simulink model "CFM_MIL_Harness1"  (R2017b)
settings: Solver=FixedStepDiscrete  StartTime=0.0  StopTime=14  FixedStep=0.01  RelTol=1e-3  EnableMultiTasking=on
undefined symbols (not defined in the file): sigbuilder_block
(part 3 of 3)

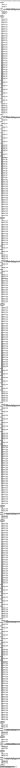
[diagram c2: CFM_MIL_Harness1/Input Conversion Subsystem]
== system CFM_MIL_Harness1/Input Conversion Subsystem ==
  note: This subsystem has been inserted by Simulink to adapt the output of the source blocks to the interface required by the harnessed component. Modifying the contents of this subsystem may result in compilation and simulation failure.
  Inport_1 : Inport
  Inport_2 : Inport  Port=2
  Inport_3 : Inport  Port=3
  Inport_4 : Inport  Port=4
  Inport_5 : Inport  Port=5
  Inport_6 : Inport  Port=6
  Inport_7 : Inport  Port=7
  Inport_8 : Inport  Port=8
  Inport_9 : Inport  Port=9
  Inport_10 : Inport  Port=10
  Inport_11 : Inport  Port=11
  Inport_12 : Inport  Port=12
  Inport_13 : Inport  Port=13
  Inport_14 : Inport  Port=14
  Inport_15 : Inport  Port=15
  Inport_16 : Inport  Port=16
  Inport_17 : Inport  Port=17
  Inport_18 : Inport  Port=18
  Inport_19 : Inport  Port=19
  Inport_20 : Inport  Port=20
  Inport_21 : Inport  Port=21
  Inport_22 : Inport  Port=22
  Inport_23 : Inport  Port=23
  Inport_24 : Inport  Port=24
  Inport_25 : Inport  Port=25
  Inport_26 : Inport  Port=26
  Inport_27 : Inport  Port=27
  Inport_28 : Inport  Port=28
  Inport_29 : Inport  Port=29
  Inport_30 : Inport  Port=30
  Inport_31 : Inport  Port=31
  Inport_32 : Inport  Port=32
  Inport_33 : Inport  Port=33
  Inport_34 : Inport  Port=34
  Inport_35 : Inport  Port=35
  Inport_36 : Inport  Port=36
  Inport_37 : Inport  Port=37
  Inport_38 : Inport  Port=38
  Inport_39 : Inport  Port=39
  Inport_40 : Inport  Port=40
  Inport_41 : Inport  Port=41
  Inport_42 : Inport  Port=42
  Inport_43 : Inport  Port=43
  Inport_44 : Inport  Port=44
  Inport_45 : Inport  Port=45
  Inport_46 : Inport  Port=46
  Inport_47 : Inport  Port=47
  Inport_48 : Inport  Port=48
  Inport_49 : Inport  Port=49
  Inport_50 : Inport  Port=50
  Inport_51 : Inport  Port=51
  Inport_52 : Inport  Port=52
  Inport_53 : Inport  Port=53
  Inport_54 : Inport  Port=54
  Inport_55 : Inport  Port=55
  Inport_56 : Inport  Port=56
  Inport_57 : Inport  Port=57
  Inport_58 : Inport  Port=58
  Inport_59 : Inport  Port=59
  Inport_60 : Inport  Port=60
  Inport_61 : Inport  Port=61
  Inport_62 : Inport  Port=62
  Inport_63 : Inport  Port=63
  Inport_64 : Inport  Port=64
  Inport_65 : Inport  Port=65
  Inport_66 : Inport  Port=66
  Inport_67 : Inport  Port=67
  Inport_68 : Inport  Port=68
  Inport_69 : Inport  Port=69
  Inport_70 : Inport  Port=70
  Inport_71 : Inport  Port=71
  Inport_72 : Inport  Port=72
  Inport_73 : Inport  Port=73
  Inport_74 : Inport  Port=74
  Inport_75 : Inport  Port=75
  Inport_76 : Inport  Port=76
  Inport_77 : Inport  Port=77
  Inport_78 : Inport  Port=78
  Inport_79 : Inport  Port=79
  Inport_80 : Inport  Port=80
  Inport_81 : Inport  Port=81
  Inport_82 : Inport  Port=82
  Inport_83 : Inport  Port=83
  Inport_84 : Inport  Port=84
  Inport_85 : Inport  Port=85
  Inport_86 : Inport  Port=86
  Inport_87 : Inport  Port=87
  Inport_88 : Inport  Port=88
  Inport_89 : Inport  Port=89
  Inport_90 : Inport  Port=90
  Inport_91 : Inport  Port=91
  Inport_92 : Inport  Port=92
  Inport_93 : Inport  Port=93
  Inport_94 : Inport  Port=94
  Inport_95 : Inport  Port=95
  Inport_96 : Inport  Port=96
  Inport_97 : Inport  Port=97
  Inport_98 : Inport  Port=98
  Inport_99 : Inport  Port=99
  Inport_100 : Inport  Port=100
  Inport_101 : Inport  Port=101
  Inport_102 : Inport  Port=102
  Inport_103 : Inport  Port=103
  Inport_104 : Inport  Port=104
  Inport_105 : Inport  Port=105
  Inport_106 : Inport  Port=106
  Inport_107 : Inport  Port=107
  Inport_108 : Inport  Port=108
  Inport_109 : Inport  Port=109
  Inport_110 : Inport  Port=110
  Inport_111 : Inport  Port=111
  Inport_112 : Inport  Port=112
  Inport_113 : Inport  Port=113
  Inport_114 : Inport  Port=114
  Inport_115 : Inport  Port=115
  Inport_116 : Inport  Port=116
  Inport_117 : Inport  Port=117
  Inport_118 : Inport  Port=118
  Inport_119 : Inport  Port=119
  Inport_120 : Inport  Port=120
  Inport_121 : Inport  Port=121
  Inport_122 : Inport  Port=122
  Inport_123 : Inport  Port=123
  Inport_124 : Inport  Port=124
  Inport_125 : Inport  Port=125
  Inport_126 : Inport  Port=126
  Inport_127 : Inport  Port=127
  Inport_128 : Inport  Port=128
  Inport_129 : Inport  Port=129
  Inport_130 : Inport  Port=130
  Inport_131 : Inport  Port=131
  Inport_132 : Inport  Port=132
  Inport_133 : Inport  Port=133
  Inport_134 : Inport  Port=134
  Inport_135 : Inport  Port=135
  Inport_136 : Inport  Port=136
  Inport_137 : Inport  Port=137
  Inport_138 : Inport  Port=138
  Inport_139 : Inport  Port=139
  Inport_140 : Inport  Port=140
  Inport_141 : Inport  Port=141
  Inport_142 : Inport  Port=142
  Inport_143 : Inport  Port=143
  Inport_144 : Inport  Port=144
  Inport_145 : Inport  Port=145
  Inport_146 : Inport  Port=146
  Inport_147 : Inport  Port=147
  Inport_148 : Inport  Port=148
  Inport_149 : Inport  Port=149
  Inport_150 : Inport  Port=150
  Inport_151 : Inport  Port=151
  Inport_152 : Inport  Port=152
  Inport_153 : Inport  Port=153
  Inport_154 : Inport  Port=154
  Inport_155 : Inport  Port=155
  Inport_156 : Inport  Port=156
  Inport_157 : Inport  Port=157
  Inport_158 : Inport  Port=158
  Inport_159 : Inport  Port=159
  Inport_160 : Inport  Port=160
  Inport_161 : Inport  Port=161
  Inport_162 : Inport  Port=162
  Inport_163 : Inport  Port=163
  Inport_164 : Inport  Port=164
  Inport_165 : Inport  Port=165
  Inport_166 : Inport  Port=166
  Inport_167 : Inport  Port=167
  Inport_168 : Inport  Port=168
  Inport_169 : Inport  Port=169
  Inport_170 : Inport  Port=170
  Inport_171 : Inport  Port=171
  Inport_172 : Inport  Port=172
  Inport_173 : Inport  Port=173
  Inport_174 : Inport  Port=174
  Inport_175 : Inport  Port=175
  Inport_176 : Inport  Port=176
  Inport_177 : Inport  Port=177
  Inport_178 : Inport  Port=178
  Inport_179 : Inport  Port=179
  Inport_180 : Inport  Port=180
  Inport_181 : Inport  Port=181
  Inport_182 : Inport  Port=182
  Inport_183 : Inport  Port=183
  Inport_184 : Inport  Port=184
  Inport_185 : Inport  Port=185
  Inport_186 : Inport  Port=186
  Inport_187 : Inport  Port=187
  Inport_188 : Inport  Port=188
  Inport_189 : Inport  Port=189
  Inport_190 : Inport  Port=190
  Inport_191 : Inport  Port=191
  Inport_192 : Inport  Port=192
  Inport_193 : Inport  Port=193
  Inport_194 : Inport  Port=194
  Inport_195 : Inport  Port=195
  Inport_196 : Inport  Port=196
  Inport_197 : Inport  Port=197
  Inport_198 : Inport  Port=198
  Inport_199 : Inport  Port=199
  Inport_200 : Inport  Port=200
  Inport_201 : Inport  Port=201
  Inport_202 : Inport  Port=202
  Inport_203 : Inport  Port=203
  Inport_204 : Inport  Port=204
  Inport_205 : Inport  Port=205
  Inport_206 : Inport  Port=206
  Inport_207 : Inport  Port=207
  Inport_208 : Inport  Port=208
  Inport_209 : Inport  Port=209
  Inport_210 : Inport  Port=210
  Inport_211 : Inport  Port=211
  Inport_212 : Inport  Port=212
  Inport_213 : Inport  Port=213
  Inport_214 : Inport  Port=214
  Inport_215 : Inport  Port=215
  Inport_216 : Inport  Port=216
  Inport_217 : Inport  Port=217
  Inport_218 : Inport  Port=218
  Inport_219 : Inport  Port=219
  Inport_220 : Inport  Port=220
  Inport_221 : Inport  Port=221
  Inport_222 : Inport  Port=222
  Inport_223 : Inport  Port=223
  Inport_224 : Inport  Port=224
  Inport_225 : Inport  Port=225
  Inport_226 : Inport  Port=226
  Inport_227 : Inport  Port=227
  Inport_228 : Inport  Port=228
  Inport_229 : Inport  Port=229
  Inport_230 : Inport  Port=230
  Inport_231 : Inport  Port=231
  Inport_232 : Inport  Port=232
  Inport_233 : Inport  Port=233
  Inport_234 : Inport  Port=234
  Inport_235 : Inport  Port=235
  Inport_236 : Inport  Port=236
  Inport_237 : Inport  Port=237
  Inport_238 : Inport  Port=238
  Inport_239 : Inport  Port=239
  Inport_240 : Inport  Port=240
  Inport_241 : Inport  Port=241
  Inport_242 : Inport  Port=242
  Inport_243 : Inport  Port=243
  Inport_244 : Inport  Port=244
  Inport_245 : Inport  Port=245
  Inport_246 : Inport  Port=246
  Inport_247 : Inport  Port=247
  Inport_248 : Inport  Port=248
  Inport_249 : Inport  Port=249
  Inport_250 : Inport  Port=250
  Inport_251 : Inport  Port=251
  Inport_252 : Inport  Port=252
  Inport_253 : Inport  Port=253
  Inport_254 : Inport  Port=254
  Inport_255 : Inport  Port=255
  Inport_256 : Inport  Port=256
  Inport_257 : Inport  Port=257
  Inport_258 : Inport  Port=258
  Inport_259 : Inport  Port=259
  Inport_260 : Inport  Port=260
  Inport_261 : Inport  Port=261
  Inport_262 : Inport  Port=262
  Inport_263 : Inport  Port=263
  Inport_264 : Inport  Port=264
  Inport_265 : Inport  Port=265
  Inport_266 : Inport  Port=266
  Inport_267 : Inport  Port=267
  Inport_268 : Inport  Port=268
  Inport_269 : Inport  Port=269
  Inport_270 : Inport  Port=270
  Inport_271 : Inport  Port=271
  Inport_272 : Inport  Port=272
  Inport_273 : Inport  Port=273
  Inport_274 : Inport  Port=274
  Inport_275 : Inport  Port=275
  Inport_276 : Inport  Port=276
  Inport_277 : Inport  Port=277
  Inport_278 : Inport  Port=278
  Inport_279 : Inport  Port=279
  Inport_280 : Inport  Port=280
  Inport_281 : Inport  Port=281
  Inport_282 : Inport  Port=282
  Inport_283 : Inport  Port=283
  Inport_284 : Inport  Port=284
  Inport_285 : Inport  Port=285
  Inport_286 : Inport  Port=286
  Inport_287 : Inport  Port=287
  Inport_288 : Inport  Port=288
  Inport_289 : Inport  Port=289
  Inport_290 : Inport  Port=290
  Inport_291 : Inport  Port=291
  Inport_292 : Inport  Port=292
  Inport_293 : Inport  Port=293
  Inport_294 : Inport  Port=294
  Inport_295 : Inport  Port=295
  Inport_296 : Inport  Port=296
  Inport_297 : Inport  Port=297
  Inport_298 : Inport  Port=298
  Inport_299 : Inport  Port=299
  Inport_300 : Inport  Port=300
  Inport_301 : Inport  Port=301
  Inport_302 : Inport  Port=302
  Inport_303 : Inport  Port=303
  Inport_304 : Inport  Port=304
  Inport_305 : Inport  Port=305
  Inport_306 : Inport  Port=306
  Inport_307 : Inport  Port=307
  Inport_308 : Inport  Port=308
  Inport_309 : Inport  Port=309
  Inport_310 : Inport  Port=310
  Inport_311 : Inport  Port=311
  Inport_312 : Inport  Port=312
  Inport_313 : Inport  Port=313
  Inport_314 : Inport  Port=314
  Inport_315 : Inport  Port=315
  Inport_316 : Inport  Port=316
  Inport_317 : Inport  Port=317
  Inport_318 : Inport  Port=318
  Inport_319 : Inport  Port=319
  Inport_320 : Inport  Port=320
  Inport_321 : Inport  Port=321
  Inport_322 : Inport  Port=322
  Inport_323 : Inport  Port=323
  Inport_324 : Inport  Port=324
  Inport_325 : Inport  Port=325
  Inport_326 : Inport  Port=326
  Inport_327 : Inport  Port=327
  Inport_328 : Inport  Port=328
  Inport_329 : Inport  Port=329
  Inport_330 : Inport  Port=330
  Inport_331 : Inport  Port=331
  Inport_332 : Inport  Port=332
  Inport_333 : Inport  Port=333
  Inport_334 : Inport  Port=334
  Inport_335 : Inport  Port=335
  Inport_336 : Inport  Port=336
  Inport_337 : Inport  Port=337
  Inport_338 : Inport  Port=338
  Inport_339 : Inport  Port=339
  Inport_340 : Inport  Port=340
  Inport_341 : Inport  Port=341
  Inport_342 : Inport  Port=342
  Inport_343 : Inport  Port=343
  Inport_344 : Inport  Port=344
  Inport_345 : Inport  Port=345
  Inport_346 : Inport  Port=346
  Inport_347 : Inport  Port=347
  Inport_348 : Inport  Port=348
  Inport_349 : Inport  Port=349
  Inport_350 : Inport  Port=350
  Inport_351 : Inport  Port=351
  Inport_352 : Inport  Port=352
  Inport_353 : Inport  Port=353
  Inport_354 : Inport  Port=354
  Inport_355 : Inport  Port=355
  Inport_356 : Inport  Port=356
  Inport_357 : Inport  Port=357
  Inport_358 : Inport  Port=358
  Inport_359 : Inport  Port=359
  Inport_360 : Inport  Port=360
  Inport_361 : Inport  Port=361
  Inport_362 : Inport  Port=362
  Inport_363 : Inport  Port=363
  Inport_364 : Inport  Port=364
  Inport_365 : Inport  Port=365
  Inport_366 : Inport  Port=366
  Inport_367 : Inport  Port=367
  Inport_368 : Inport  Port=368
  Inport_369 : Inport  Port=369
  Inport_370 : Inport  Port=370
  Inport_371 : Inport  Port=371
  Inport_372 : Inport  Port=372
  Inport_373 : Inport  Port=373
  Inport_374 : Inport  Port=374
  Inport_375 : Inport  Port=375
  Inport_376 : Inport  Port=376
  Inport_377 : Inport  Port=377
  Inport_378 : Inport  Port=378
  Inport_379 : Inport  Port=379
  Inport_380 : Inport  Port=380
  Inport_381 : Inport  Port=381
  Inport_382 : Inport  Port=382
  Inport_383 : Inport  Port=383
  Inport_384 : Inport  Port=384
  Inport_385 : Inport  Port=385
  Inport_386 : Inport  Port=386
  Inport_387 : Inport  Port=387
  Inport_388 : Inport  Port=388
  Inport_389 : Inport  Port=389
  Inport_390 : Inport  Port=390
  Inport_391 : Inport  Port=391
  Inport_392 : Inport  Port=392
  Inport_393 : Inport  Port=393
  Inport_394 : Inport  Port=394
  Inport_395 : Inport  Port=395
  Inport_396 : Inport  Port=396
  Inport_397 : Inport  Port=397
  Inport_398 : Inport  Port=398
  Inport_399 : Inport  Port=399
  Inport_400 : Inport  Port=400
  Inport_401 : Inport  Port=401
  Inport_402 : Inport  Port=402
  Inport_403 : Inport  Port=403
  Inport_404 : Inport  Port=404
  Inport_405 : Inport  Port=405
  Inport_406 : Inport  Port=406
  Inport_407 : Inport  Port=407
  Inport_408 : Inport  Port=408
  Inport_409 : Inport  Port=409
  Inport_410 : Inport  Port=410
  Inport_411 : Inport  Port=411
  Inport_412 : Inport  Port=412
  Inport_413 : Inport  Port=413
  Inport_414 : Inport  Port=414
  Inport_415 : Inport  Port=415
  Inport_416 : Inport  Port=416
  Inport_417 : Inport  Port=417
  Inport_418 : Inport  Port=418
  Inport_419 : Inport  Port=419
  Inport_420 : Inport  Port=420
  Inport_421 : Inport  Port=421
  Inport_422 : Inport  Port=422
  Inport_423 : Inport  Port=423
  Inport_424 : Inport  Port=424
  Inport_425 : Inport  Port=425
  Concat_{1,5,7..9} (5 alike) : Concatenate  NumInputs=8
  Concat_2 : Concatenate  NumInputs=112
  Concat_3 : Concatenate  NumInputs=48
  Concat_4 : Concatenate  NumInputs=112
  Concat_6 : Concatenate  NumInputs=112
  Data_Conversion_{1,3,5,7,11,13,19} (7 alike) : DataTypeConversion  OutDataTypeStr=uint8
  Data_Conversion_{2,10,14,16,18} (5 alike) : Reshape  OutputDimensionality=Customize  OutputDimensions=[8]
  Data_Conversion_12 : Reshape  OutputDimensionality=Customize  OutputDimensions=[112]
  Data_Conversion_15 : DataTypeConversion  OutDataTypeStr=uint16
  Data_Conversion_17 : DataTypeConversion  OutDataTypeStr=uint16
  Data_Conversion_4 : Reshape  OutputDimensionality=Customize  OutputDimensions=[112]
  Data_Conversion_6 : Reshape  OutputDimensionality=Customize  OutputDimensions=[48]
  Data_Conversion_8 : Reshape  OutputDimensionality=Customize  OutputDimensions=[112]
  Data_Conversion_9 : DataTypeConversion  OutDataTypeStr=boolean
  RateTs_{1..10} (10 alike) : RateTransition  OutPortSampleTime=0.01
  SigSpec_1 : SignalSpecification  OutDataTypeStr=uint8  Unit=numb  Dimensions=[8]  SampleTime=0.01
  SigSpec_10 : SignalSpecification  OutDataTypeStr=uint8  Unit=numb  Dimensions=[1]  SampleTime=0.01
  SigSpec_2 : SignalSpecification  OutDataTypeStr=uint8  Unit=numb  Dimensions=[112]  SampleTime=0.01
  SigSpec_3 : SignalSpecification  OutDataTypeStr=uint8  Unit=numb  Dimensions=[48]  SampleTime=0.01
  SigSpec_4 : SignalSpecification  OutDataTypeStr=uint8  Unit=numb  Dimensions=[112]  SampleTime=0.01
  SigSpec_5 : SignalSpecification  OutDataTypeStr=boolean  Unit=flag  Dimensions=[8]  SampleTime=0.01
  SigSpec_6 : SignalSpecification  OutDataTypeStr=uint8  Unit=numb  Dimensions=[112]  SampleTime=0.01
  SigSpec_7 : SignalSpecification  OutDataTypeStr=uint8  Unit=numb  Dimensions=[8]  SampleTime=0.01
  SigSpec_8 : SignalSpecification  OutDataTypeStr=uint16  Unit=numb  Dimensions=[8]  SampleTime=0.01
  SigSpec_9 : SignalSpecification  OutDataTypeStr=uint16  Unit=numb  Dimensions=[8]  SampleTime=0.01
  Outport_1 : Outport
  Outport_2 : Outport  Port=2
  Outport_3 : Outport  Port=3
  Outport_4 : Outport  Port=4
  Outport_5 : Outport  Port=5
  Outport_6 : Outport  Port=6
  Outport_7 : Outport  Port=7
  Outport_8 : Outport  Port=8
  Outport_9 : Outport  Port=9
  Outport_10 : Outport  Port=10
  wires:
  SigSpec_1/1 -> Outport_1/1
  RateTs_1/1 -> SigSpec_1/1
  Data_Conversion_1/1 -> RateTs_1/1
  Data_Conversion_2/1 -> Data_Conversion_1/1
  Concat_1/1 -> Data_Conversion_2/1
  Inport_1/1 -> Concat_1/1
  Inport_2/1 -> Concat_1/2
  Inport_3/1 -> Concat_1/3
  Inport_4/1 -> Concat_1/4
  Inport_5/1 -> Concat_1/5
  Inport_6/1 -> Concat_1/6
  Inport_7/1 -> Concat_1/7
  Inport_8/1 -> Concat_1/8
  SigSpec_2/1 -> Outport_2/1
  RateTs_2/1 -> SigSpec_2/1
  Data_Conversion_3/1 -> RateTs_2/1
  Data_Conversion_4/1 -> Data_Conversion_3/1
  Concat_2/1 -> Data_Conversion_4/1
  Inport_9/1 -> Concat_2/1
  Inport_10/1 -> Concat_2/2
  Inport_11/1 -> Concat_2/3
  Inport_12/1 -> Concat_2/4
  Inport_13/1 -> Concat_2/5
  Inport_14/1 -> Concat_2/6
  Inport_15/1 -> Concat_2/7
  Inport_16/1 -> Concat_2/8
  Inport_17/1 -> Concat_2/9
  Inport_18/1 -> Concat_2/10
  Inport_19/1 -> Concat_2/11
  Inport_20/1 -> Concat_2/12
  Inport_21/1 -> Concat_2/13
  Inport_22/1 -> Concat_2/14
  Inport_23/1 -> Concat_2/15
  Inport_24/1 -> Concat_2/16
  Inport_25/1 -> Concat_2/17
  Inport_26/1 -> Concat_2/18
  Inport_27/1 -> Concat_2/19
  Inport_28/1 -> Concat_2/20
  Inport_29/1 -> Concat_2/21
  Inport_30/1 -> Concat_2/22
  Inport_31/1 -> Concat_2/23
  Inport_32/1 -> Concat_2/24
  Inport_33/1 -> Concat_2/25
  Inport_34/1 -> Concat_2/26
  Inport_35/1 -> Concat_2/27
  Inport_36/1 -> Concat_2/28
  Inport_37/1 -> Concat_2/29
  Inport_38/1 -> Concat_2/30
  Inport_39/1 -> Concat_2/31
  Inport_40/1 -> Concat_2/32
  Inport_41/1 -> Concat_2/33
  Inport_42/1 -> Concat_2/34
  Inport_43/1 -> Concat_2/35
  Inport_44/1 -> Concat_2/36
  Inport_45/1 -> Concat_2/37
  Inport_46/1 -> Concat_2/38
  Inport_47/1 -> Concat_2/39
  Inport_48/1 -> Concat_2/40
  Inport_49/1 -> Concat_2/41
  Inport_50/1 -> Concat_2/42
  Inport_51/1 -> Concat_2/43
  Inport_52/1 -> Concat_2/44
  Inport_53/1 -> Concat_2/45
  Inport_54/1 -> Concat_2/46
  Inport_55/1 -> Concat_2/47
  Inport_56/1 -> Concat_2/48
  Inport_57/1 -> Concat_2/49
  Inport_58/1 -> Concat_2/50
  Inport_59/1 -> Concat_2/51
  Inport_60/1 -> Concat_2/52
  Inport_61/1 -> Concat_2/53
  Inport_62/1 -> Concat_2/54
  Inport_63/1 -> Concat_2/55
  Inport_64/1 -> Concat_2/56
  Inport_65/1 -> Concat_2/57
  Inport_66/1 -> Concat_2/58
  Inport_67/1 -> Concat_2/59
  Inport_68/1 -> Concat_2/60
  Inport_69/1 -> Concat_2/61
  Inport_70/1 -> Concat_2/62
  Inport_71/1 -> Concat_2/63
  Inport_72/1 -> Concat_2/64
  Inport_73/1 -> Concat_2/65
  Inport_74/1 -> Concat_2/66
  Inport_75/1 -> Concat_2/67
  Inport_76/1 -> Concat_2/68
  Inport_77/1 -> Concat_2/69
  Inport_78/1 -> Concat_2/70
  Inport_79/1 -> Concat_2/71
  Inport_80/1 -> Concat_2/72
  Inport_81/1 -> Concat_2/73
  Inport_82/1 -> Concat_2/74
  Inport_83/1 -> Concat_2/75
  Inport_84/1 -> Concat_2/76
  Inport_85/1 -> Concat_2/77
  Inport_86/1 -> Concat_2/78
  Inport_87/1 -> Concat_2/79
  Inport_88/1 -> Concat_2/80
  Inport_89/1 -> Concat_2/81
  Inport_90/1 -> Concat_2/82
  Inport_91/1 -> Concat_2/83
  Inport_92/1 -> Concat_2/84
  Inport_93/1 -> Concat_2/85
  Inport_94/1 -> Concat_2/86
  Inport_95/1 -> Concat_2/87
  Inport_96/1 -> Concat_2/88
  Inport_97/1 -> Concat_2/89
  Inport_98/1 -> Concat_2/90
  Inport_99/1 -> Concat_2/91
  Inport_100/1 -> Concat_2/92
  Inport_101/1 -> Concat_2/93
  Inport_102/1 -> Concat_2/94
  Inport_103/1 -> Concat_2/95
  Inport_104/1 -> Concat_2/96
  Inport_105/1 -> Concat_2/97
  Inport_106/1 -> Concat_2/98
  Inport_107/1 -> Concat_2/99
  Inport_108/1 -> Concat_2/100
  Inport_109/1 -> Concat_2/101
  Inport_110/1 -> Concat_2/102
  Inport_111/1 -> Concat_2/103
  Inport_112/1 -> Concat_2/104
  Inport_113/1 -> Concat_2/105
  Inport_114/1 -> Concat_2/106
  Inport_115/1 -> Concat_2/107
  Inport_116/1 -> Concat_2/108
  Inport_117/1 -> Concat_2/109
  Inport_118/1 -> Concat_2/110
  Inport_119/1 -> Concat_2/111
  Inport_120/1 -> Concat_2/112
  SigSpec_3/1 -> Outport_3/1
  RateTs_3/1 -> SigSpec_3/1
  Data_Conversion_5/1 -> RateTs_3/1
  Data_Conversion_6/1 -> Data_Conversion_5/1
  Concat_3/1 -> Data_Conversion_6/1
  Inport_121/1 -> Concat_3/1
  Inport_122/1 -> Concat_3/2
  Inport_123/1 -> Concat_3/3
  Inport_124/1 -> Concat_3/4
  Inport_125/1 -> Concat_3/5
  Inport_126/1 -> Concat_3/6
  Inport_127/1 -> Concat_3/7
  Inport_128/1 -> Concat_3/8
  Inport_129/1 -> Concat_3/9
  Inport_130/1 -> Concat_3/10
  Inport_131/1 -> Concat_3/11
  Inport_132/1 -> Concat_3/12
  Inport_133/1 -> Concat_3/13
  Inport_134/1 -> Concat_3/14
  Inport_135/1 -> Concat_3/15
  Inport_136/1 -> Concat_3/16
  Inport_137/1 -> Concat_3/17
  Inport_138/1 -> Concat_3/18
  Inport_139/1 -> Concat_3/19
  Inport_140/1 -> Concat_3/20
  Inport_141/1 -> Concat_3/21
  Inport_142/1 -> Concat_3/22
  Inport_143/1 -> Concat_3/23
  Inport_144/1 -> Concat_3/24
  Inport_145/1 -> Concat_3/25
  Inport_146/1 -> Concat_3/26
  Inport_147/1 -> Concat_3/27
  Inport_148/1 -> Concat_3/28
  Inport_149/1 -> Concat_3/29
  Inport_150/1 -> Concat_3/30
  Inport_151/1 -> Concat_3/31
  Inport_152/1 -> Concat_3/32
  Inport_153/1 -> Concat_3/33
  Inport_154/1 -> Concat_3/34
  Inport_155/1 -> Concat_3/35
  Inport_156/1 -> Concat_3/36
  Inport_157/1 -> Concat_3/37
  Inport_158/1 -> Concat_3/38
  Inport_159/1 -> Concat_3/39
  Inport_160/1 -> Concat_3/40
  Inport_161/1 -> Concat_3/41
  Inport_162/1 -> Concat_3/42
  Inport_163/1 -> Concat_3/43
  Inport_164/1 -> Concat_3/44
  Inport_165/1 -> Concat_3/45
  Inport_166/1 -> Concat_3/46
  Inport_167/1 -> Concat_3/47
  Inport_168/1 -> Concat_3/48
  SigSpec_4/1 -> Outport_4/1
  RateTs_4/1 -> SigSpec_4/1
  Data_Conversion_7/1 -> RateTs_4/1
  Data_Conversion_8/1 -> Data_Conversion_7/1
  Concat_4/1 -> Data_Conversion_8/1
  Inport_169/1 -> Concat_4/1
  Inport_170/1 -> Concat_4/2
  Inport_171/1 -> Concat_4/3
  Inport_172/1 -> Concat_4/4
  Inport_173/1 -> Concat_4/5
  Inport_174/1 -> Concat_4/6
  Inport_175/1 -> Concat_4/7
  Inport_176/1 -> Concat_4/8
  Inport_177/1 -> Concat_4/9
  Inport_178/1 -> Concat_4/10
  Inport_179/1 -> Concat_4/11
  Inport_180/1 -> Concat_4/12
  Inport_181/1 -> Concat_4/13
  Inport_182/1 -> Concat_4/14
  Inport_183/1 -> Concat_4/15
  Inport_184/1 -> Concat_4/16
  Inport_185/1 -> Concat_4/17
  Inport_186/1 -> Concat_4/18
  Inport_187/1 -> Concat_4/19
  Inport_188/1 -> Concat_4/20
  Inport_189/1 -> Concat_4/21
  Inport_190/1 -> Concat_4/22
  Inport_191/1 -> Concat_4/23
  Inport_192/1 -> Concat_4/24
  Inport_193/1 -> Concat_4/25
  Inport_194/1 -> Concat_4/26
  Inport_195/1 -> Concat_4/27
  Inport_196/1 -> Concat_4/28
  Inport_197/1 -> Concat_4/29
  Inport_198/1 -> Concat_4/30
  Inport_199/1 -> Concat_4/31
  Inport_200/1 -> Concat_4/32
  Inport_201/1 -> Concat_4/33
  Inport_202/1 -> Concat_4/34
  Inport_203/1 -> Concat_4/35
  Inport_204/1 -> Concat_4/36
  Inport_205/1 -> Concat_4/37
  Inport_206/1 -> Concat_4/38
  Inport_207/1 -> Concat_4/39
  Inport_208/1 -> Concat_4/40
  Inport_209/1 -> Concat_4/41
  Inport_210/1 -> Concat_4/42
  Inport_211/1 -> Concat_4/43
  Inport_212/1 -> Concat_4/44
  Inport_213/1 -> Concat_4/45
  Inport_214/1 -> Concat_4/46
  Inport_215/1 -> Concat_4/47
  Inport_216/1 -> Concat_4/48
  Inport_217/1 -> Concat_4/49
  Inport_218/1 -> Concat_4/50
  Inport_219/1 -> Concat_4/51
  Inport_220/1 -> Concat_4/52
  Inport_221/1 -> Concat_4/53
  Inport_222/1 -> Concat_4/54
  Inport_223/1 -> Concat_4/55
  Inport_224/1 -> Concat_4/56
  Inport_225/1 -> Concat_4/57
  Inport_226/1 -> Concat_4/58
  Inport_227/1 -> Concat_4/59
  Inport_228/1 -> Concat_4/60
  Inport_229/1 -> Concat_4/61
  Inport_230/1 -> Concat_4/62
  Inport_231/1 -> Concat_4/63
  Inport_232/1 -> Concat_4/64
  Inport_233/1 -> Concat_4/65
  Inport_234/1 -> Concat_4/66
  Inport_235/1 -> Concat_4/67
  Inport_236/1 -> Concat_4/68
  Inport_237/1 -> Concat_4/69
  Inport_238/1 -> Concat_4/70
  Inport_239/1 -> Concat_4/71
  Inport_240/1 -> Concat_4/72
  Inport_241/1 -> Concat_4/73
  Inport_242/1 -> Concat_4/74
  Inport_243/1 -> Concat_4/75
  Inport_244/1 -> Concat_4/76
  Inport_245/1 -> Concat_4/77
  Inport_246/1 -> Concat_4/78
  Inport_247/1 -> Concat_4/79
  Inport_248/1 -> Concat_4/80
  Inport_249/1 -> Concat_4/81
  Inport_250/1 -> Concat_4/82
  Inport_251/1 -> Concat_4/83
  Inport_252/1 -> Concat_4/84
  Inport_253/1 -> Concat_4/85
  Inport_254/1 -> Concat_4/86
  Inport_255/1 -> Concat_4/87
  Inport_256/1 -> Concat_4/88
  Inport_257/1 -> Concat_4/89
  Inport_258/1 -> Concat_4/90
  Inport_259/1 -> Concat_4/91
  Inport_260/1 -> Concat_4/92
  Inport_261/1 -> Concat_4/93
  Inport_262/1 -> Concat_4/94
  Inport_263/1 -> Concat_4/95
  Inport_264/1 -> Concat_4/96
  Inport_265/1 -> Concat_4/97
  Inport_266/1 -> Concat_4/98
  Inport_267/1 -> Concat_4/99
  Inport_268/1 -> Concat_4/100
  Inport_269/1 -> Concat_4/101
  Inport_270/1 -> Concat_4/102
  Inport_271/1 -> Concat_4/103
  Inport_272/1 -> Concat_4/104
  Inport_273/1 -> Concat_4/105
  Inport_274/1 -> Concat_4/106
  Inport_275/1 -> Concat_4/107
  Inport_276/1 -> Concat_4/108
  Inport_277/1 -> Concat_4/109
  Inport_278/1 -> Concat_4/110
  Inport_279/1 -> Concat_4/111
  Inport_280/1 -> Concat_4/112
  SigSpec_5/1 -> Outport_5/1
  RateTs_5/1 -> SigSpec_5/1
  Data_Conversion_9/1 -> RateTs_5/1
  Data_Conversion_10/1 -> Data_Conversion_9/1
  Concat_5/1 -> Data_Conversion_10/1
  Inport_281/1 -> Concat_5/1
  Inport_282/1 -> Concat_5/2
  Inport_283/1 -> Concat_5/3
  Inport_284/1 -> Concat_5/4
  Inport_285/1 -> Concat_5/5
  Inport_286/1 -> Concat_5/6
  Inport_287/1 -> Concat_5/7
  Inport_288/1 -> Concat_5/8
  SigSpec_6/1 -> Outport_6/1
  RateTs_6/1 -> SigSpec_6/1
  Data_Conversion_11/1 -> RateTs_6/1
  Data_Conversion_12/1 -> Data_Conversion_11/1
  Concat_6/1 -> Data_Conversion_12/1
  Inport_289/1 -> Concat_6/1
  Inport_290/1 -> Concat_6/2
  Inport_291/1 -> Concat_6/3
  Inport_292/1 -> Concat_6/4
  Inport_293/1 -> Concat_6/5
  Inport_294/1 -> Concat_6/6
  Inport_295/1 -> Concat_6/7
  Inport_296/1 -> Concat_6/8
  Inport_297/1 -> Concat_6/9
  Inport_298/1 -> Concat_6/10
  Inport_299/1 -> Concat_6/11
  Inport_300/1 -> Concat_6/12
  Inport_301/1 -> Concat_6/13
  Inport_302/1 -> Concat_6/14
  Inport_303/1 -> Concat_6/15
  Inport_304/1 -> Concat_6/16
  Inport_305/1 -> Concat_6/17
  Inport_306/1 -> Concat_6/18
  Inport_307/1 -> Concat_6/19
  Inport_308/1 -> Concat_6/20
  Inport_309/1 -> Concat_6/21
  Inport_310/1 -> Concat_6/22
  Inport_311/1 -> Concat_6/23
  Inport_312/1 -> Concat_6/24
  Inport_313/1 -> Concat_6/25
  Inport_314/1 -> Concat_6/26
  Inport_315/1 -> Concat_6/27
  Inport_316/1 -> Concat_6/28
  Inport_317/1 -> Concat_6/29
  Inport_318/1 -> Concat_6/30
  Inport_319/1 -> Concat_6/31
  Inport_320/1 -> Concat_6/32
  Inport_321/1 -> Concat_6/33
  Inport_322/1 -> Concat_6/34
  Inport_323/1 -> Concat_6/35
  Inport_324/1 -> Concat_6/36
  Inport_325/1 -> Concat_6/37
  Inport_326/1 -> Concat_6/38
  Inport_327/1 -> Concat_6/39
  Inport_328/1 -> Concat_6/40
  Inport_329/1 -> Concat_6/41
  Inport_330/1 -> Concat_6/42
  Inport_331/1 -> Concat_6/43
  Inport_332/1 -> Concat_6/44
  Inport_333/1 -> Concat_6/45
  Inport_334/1 -> Concat_6/46
  Inport_335/1 -> Concat_6/47
  Inport_336/1 -> Concat_6/48
  Inport_337/1 -> Concat_6/49
  Inport_338/1 -> Concat_6/50
  Inport_339/1 -> Concat_6/51
  Inport_340/1 -> Concat_6/52
  Inport_341/1 -> Concat_6/53
  Inport_342/1 -> Concat_6/54
  Inport_343/1 -> Concat_6/55
  Inport_344/1 -> Concat_6/56
  Inport_345/1 -> Concat_6/57
  Inport_346/1 -> Concat_6/58
  Inport_347/1 -> Concat_6/59
  Inport_348/1 -> Concat_6/60
  Inport_349/1 -> Concat_6/61
  Inport_350/1 -> Concat_6/62
  Inport_351/1 -> Concat_6/63
  Inport_352/1 -> Concat_6/64
  Inport_353/1 -> Concat_6/65
  Inport_354/1 -> Concat_6/66
  Inport_355/1 -> Concat_6/67
  Inport_356/1 -> Concat_6/68
  Inport_357/1 -> Concat_6/69
  Inport_358/1 -> Concat_6/70
  Inport_359/1 -> Concat_6/71
  Inport_360/1 -> Concat_6/72
  Inport_361/1 -> Concat_6/73
  Inport_362/1 -> Concat_6/74
  Inport_363/1 -> Concat_6/75
  Inport_364/1 -> Concat_6/76
  Inport_365/1 -> Concat_6/77
  Inport_366/1 -> Concat_6/78
  Inport_367/1 -> Concat_6/79
  Inport_368/1 -> Concat_6/80
  Inport_369/1 -> Concat_6/81
  Inport_370/1 -> Concat_6/82
  Inport_371/1 -> Concat_6/83
  Inport_372/1 -> Concat_6/84
  Inport_373/1 -> Concat_6/85
  Inport_374/1 -> Concat_6/86
  Inport_375/1 -> Concat_6/87
  Inport_376/1 -> Concat_6/88
  Inport_377/1 -> Concat_6/89
  Inport_378/1 -> Concat_6/90
  Inport_379/1 -> Concat_6/91
  Inport_380/1 -> Concat_6/92
  Inport_381/1 -> Concat_6/93
  Inport_382/1 -> Concat_6/94
  Inport_383/1 -> Concat_6/95
  Inport_384/1 -> Concat_6/96
  Inport_385/1 -> Concat_6/97
  Inport_386/1 -> Concat_6/98
  Inport_387/1 -> Concat_6/99
  Inport_388/1 -> Concat_6/100
  Inport_389/1 -> Concat_6/101
  Inport_390/1 -> Concat_6/102
  Inport_391/1 -> Concat_6/103
  Inport_392/1 -> Concat_6/104
  Inport_393/1 -> Concat_6/105
  Inport_394/1 -> Concat_6/106
  Inport_395/1 -> Concat_6/107
  Inport_396/1 -> Concat_6/108
  Inport_397/1 -> Concat_6/109
  Inport_398/1 -> Concat_6/110
  Inport_399/1 -> Concat_6/111
  Inport_400/1 -> Concat_6/112
  SigSpec_7/1 -> Outport_7/1
  RateTs_7/1 -> SigSpec_7/1
  Data_Conversion_13/1 -> RateTs_7/1
  Data_Conversion_14/1 -> Data_Conversion_13/1
  Concat_7/1 -> Data_Conversion_14/1
  Inport_401/1 -> Concat_7/1
  Inport_402/1 -> Concat_7/2
  Inport_403/1 -> Concat_7/3
  Inport_404/1 -> Concat_7/4
  Inport_405/1 -> Concat_7/5
  Inport_406/1 -> Concat_7/6
  Inport_407/1 -> Concat_7/7
  Inport_408/1 -> Concat_7/8
  SigSpec_8/1 -> Outport_8/1
  RateTs_8/1 -> SigSpec_8/1
  Data_Conversion_15/1 -> RateTs_8/1
  Data_Conversion_16/1 -> Data_Conversion_15/1
  Concat_8/1 -> Data_Conversion_16/1
  Inport_409/1 -> Concat_8/1
  Inport_410/1 -> Concat_8/2
  Inport_411/1 -> Concat_8/3
  Inport_412/1 -> Concat_8/4
  Inport_413/1 -> Concat_8/5
  Inport_414/1 -> Concat_8/6
  Inport_415/1 -> Concat_8/7
  Inport_416/1 -> Concat_8/8
  SigSpec_9/1 -> Outport_9/1
  RateTs_9/1 -> SigSpec_9/1
  Data_Conversion_17/1 -> RateTs_9/1
  Data_Conversion_18/1 -> Data_Conversion_17/1
  Concat_9/1 -> Data_Conversion_18/1
  Inport_417/1 -> Concat_9/1
  Inport_418/1 -> Concat_9/2
  Inport_419/1 -> Concat_9/3
  Inport_420/1 -> Concat_9/4
  Inport_421/1 -> Concat_9/5
  Inport_422/1 -> Concat_9/6
  Inport_423/1 -> Concat_9/7
  Inport_424/1 -> Concat_9/8
  SigSpec_10/1 -> Outport_10/1
  RateTs_10/1 -> SigSpec_10/1
  Data_Conversion_19/1 -> RateTs_10/1
  Inport_425/1 -> Data_Conversion_19/1

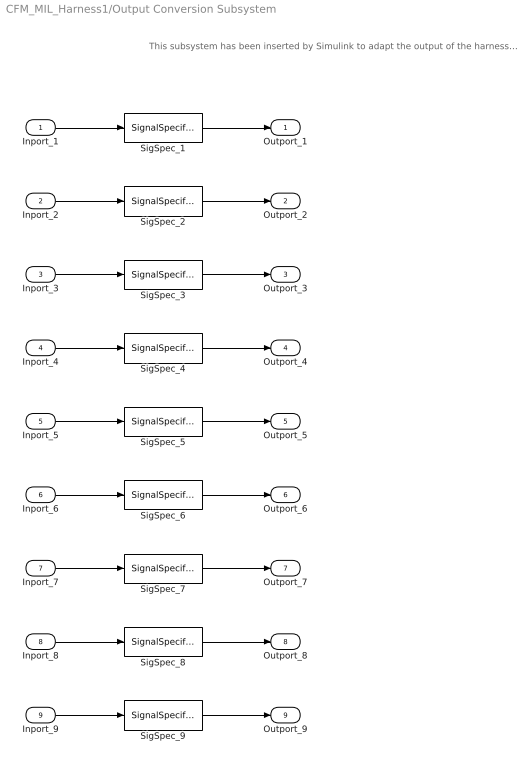
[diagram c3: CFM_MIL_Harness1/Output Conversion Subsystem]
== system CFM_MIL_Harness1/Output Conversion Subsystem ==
  note: This subsystem has been inserted by Simulink to adapt the output of the harnessed component to the interface required by the sink blocks. Modifying the contents of this subsystem may result in compilation and simulation failure.
  Inport_1 : Inport
  Inport_2 : Inport  Port=2
  Inport_3 : Inport  Port=3
  Inport_4 : Inport  Port=4
  Inport_5 : Inport  Port=5
  Inport_6 : Inport  Port=6
  Inport_7 : Inport  Port=7
  Inport_8 : Inport  Port=8
  Inport_9 : Inport  Port=9
  SigSpec_{1..9} (9 alike) : SignalSpecification  OutDataTypeStr=boolean  Unit=flg  Dimensions=[8]  SampleTime=0.01
  Outport_1 : Outport
  Outport_2 : Outport  Port=2
  Outport_3 : Outport  Port=3
  Outport_4 : Outport  Port=4
  Outport_5 : Outport  Port=5
  Outport_6 : Outport  Port=6
  Outport_7 : Outport  Port=7
  Outport_8 : Outport  Port=8
  Outport_9 : Outport  Port=9
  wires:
  Inport_1/1 -> SigSpec_1/1
  SigSpec_1/1 -> Outport_1/1
  Inport_2/1 -> SigSpec_2/1
  SigSpec_2/1 -> Outport_2/1
  Inport_3/1 -> SigSpec_3/1
  SigSpec_3/1 -> Outport_3/1
  Inport_4/1 -> SigSpec_4/1
  SigSpec_4/1 -> Outport_4/1
  Inport_5/1 -> SigSpec_5/1
  SigSpec_5/1 -> Outport_5/1
  Inport_6/1 -> SigSpec_6/1
  SigSpec_6/1 -> Outport_6/1
  Inport_7/1 -> SigSpec_7/1
  SigSpec_7/1 -> Outport_7/1
  Inport_8/1 -> SigSpec_8/1
  SigSpec_8/1 -> Outport_8/1
  Inport_9/1 -> SigSpec_9/1
  SigSpec_9/1 -> Outport_9/1
